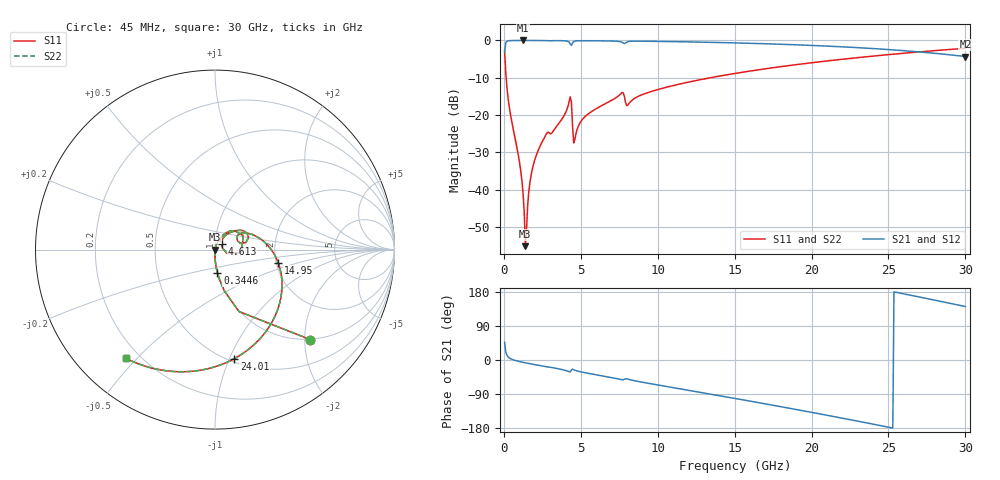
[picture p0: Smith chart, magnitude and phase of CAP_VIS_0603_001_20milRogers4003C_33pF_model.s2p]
! S-parameter model data by Modelithics Inc.  support@modelithics.com  813-866-6335  Tampa FL USA
! S-Parameter data specifications:
! Substrate: 20-mil Rogers 4003C, substrate thickness, H=0.508mm, Dielectric constant, Er=3.75
! PCB Mounting Pad Footprint: Pad width, PadW=0.90mm , Pad length, PadL=1.00mm , Pad gap, PadG (edge-to-edge)=1.00mm , Reference planes=3.0mm apart
! Created Wed Nov 18 13:28:09 2015
# hz S ma R 50
! 2 Port Network Data from SP1.SP block
! freq  magS11  angS11  magS21  angS21  magS12  angS12  magS22  angS22
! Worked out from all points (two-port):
!   401 points, 45 MHz to 30 GHz, reference 50 ohm
!   highest |S21| = -0.01 dB at 1.243 GHz (marker M1); lowest = -4.3 dB at 30 GHz (marker M2)
!   |S21| within 3 dB of the highest: 53.1 MHz to 26.8 GHz (26.75 GHz wide, 199 % of centre)
!   lowest |S11| = -55.1 dB at 1.393 GHz (marker M3), VSWR 1.00, Z = 50.1 - j0.13 ohm
!   |S11| at or under -10 dB: 145.7 MHz to 13.42 GHz (13.27 GHz wide, 196 % of centre)
!   |S22| runs from -55.1 to -2.1 dB; largest |S21 - S12| = 0
!   S11 on the Smith chart (normalised r, x): 45 MHz: 0.99, -2.12; 344.6 MHz: 0.99, -0.26; 4.613 GHz: 1.07, +0.06; 14.95 GHz: 2.05, -0.34; 24.01 GHz: 0.53, -1.04; 30 GHz: 0.15, -0.46
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4.5e7  0.7293 -43.4  0.6839 46.6  0.6839 46.6  0.7293 -43.4
3.4455e8  0.1301 -84.1  0.9908 5.6  0.9908 5.6  0.1301 -84.1
1.018538e9  0.02295 -91.2  0.9985 -4.1  0.9985 -4.1  0.02295 -91.2
1.2432e9  0.009051 -88.0  0.9986 -6.1  0.9986 -6.1  0.009051 -88.0
1.392975e9  0.001759 -47.3  0.9985 -7.4  0.9985 -7.4  0.001759 -47.3
1.54275e9  0.006114 67.9  0.9984 -8.6  0.9984 -8.6  0.006114 67.9
1.692525e9  0.01257 73.4  0.9983 -9.7  0.9983 -9.7  0.01257 73.4
1.917188e9  0.02169 74.2  0.998 -11.5  0.998 -11.5  0.02169 74.2
2.666062e9  0.05155 68.4  0.9944 -17.1  0.9944 -17.1  0.05155 68.4
3.6396e9  0.08115 62.8  0.9919 -24.0  0.9919 -24.0  0.08115 62.8
4.2387e9  0.1517 43.8  0.949 -31.0  0.949 -31.0  0.1517 43.8
4.613138e9  0.04733 38.7  0.9792 -27.0  0.9792 -27.0  0.04733 38.7
5.062462e9  0.0855 54.5  0.9905 -31.8  0.9905 -31.8  0.0855 54.5
7.608638e9  0.1945 31.2  0.956 -51.6  0.956 -51.6  0.1945 31.2
8.057962e9  0.1367 27.4  0.9617 -50.5  0.9617 -50.5  0.1367 27.4
1.007992e10  0.222 22.5  0.9698 -66.4  0.9698 -66.4  0.222 22.5
1.494761e10  0.3592 -11.6  0.9272 -100.9  0.9272 -100.9  0.3592 -11.6
1.50225e10  0.3613 -12.2  0.9263 -101.4  0.9263 -101.4  0.3613 -12.2
2.003996e10  0.5034 -49.1  0.8564 -138.4  0.8564 -138.4  0.5034 -49.1
2.4009e10  0.617 -79.9  0.7777 -169.3  0.7777 -169.3  0.617 -79.9
2.505742e10  0.647 -88.3  0.7528 -177.8  0.7528 -177.8  0.647 -88.3
3e10  0.7834 -129.4  0.6088 141.1  0.6088 141.1  0.7834 -129.4
